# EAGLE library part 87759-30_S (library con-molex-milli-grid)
HEADER
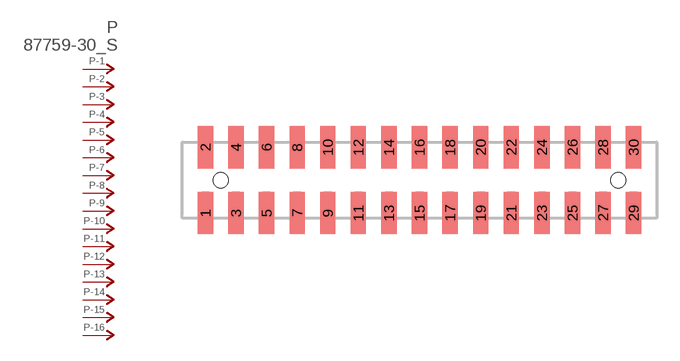
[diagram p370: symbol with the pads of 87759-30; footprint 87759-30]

Designator prefix P; gates -1=P-NV -2=P-N -3=P-N -4=P-N -5=P-N -6=P-N -7=P-N -8=P-N -9=P-N -10=P-N -11=P-N -12=P-N -13=P-N -14=P-N -15=P-N -16=P-N -17=P-N -18=P-N -19=P-N -20=P-N -21=P-N -22=P-N -23=P-N -24=P-N -25=P-N -26=P-N -27=P-N -28=P-N -29=P-N -30=P-N

## 87759-30_S  [87759-30]
1  -1:P  pas
2  -2:P  pas
3  -3:P  pas
4  -4:P  pas
5  -5:P  pas
6  -6:P  pas
7  -7:P  pas
8  -8:P  pas
9  -9:P  pas
10  -10:P  pas
11  -11:P  pas
12  -12:P  pas
13  -13:P  pas
14  -14:P  pas
15  -15:P  pas
16  -16:P  pas
17  -17:P  pas
18  -18:P  pas
19  -19:P  pas
20  -20:P  pas
21  -21:P  pas
22  -22:P  pas
23  -23:P  pas
24  -24:P  pas
25  -25:P  pas
26  -26:P  pas
27  -27:P  pas
28  -28:P  pas
29  -29:P  pas
30  -30:P  pas

## Footprint 87759-30 (pad centres in mm)
HEADER SMD Dual Row, Vertical
smd 1 x 2.75: 1 -14,-2.15; 2 -14,2.15; 3 -12,-2.15; 4 -12,2.15; 5 -10,-2.15; 6 -10,2.15; 7 -8,-2.15; 8 -8,2.15; 9 -6,-2.15; 10 -6,2.15; 11 -4,-2.15; 12 -4,2.15; 13 -2,-2.15; 14 -2,2.15; 15 0,-2.15; 16 0,2.15; 17 2,-2.15; 18 2,2.15; 19 4,-2.15; 20 4,2.15; 21 6,-2.15; 22 6,2.15; 23 8,-2.15; 24 8,2.15; 25 10,-2.15; 26 10,2.15; 27 12,-2.15; 28 12,2.15; 29 14,-2.15; 30 14,2.15
hole 1 at -13,0
hole 1 at 13,0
